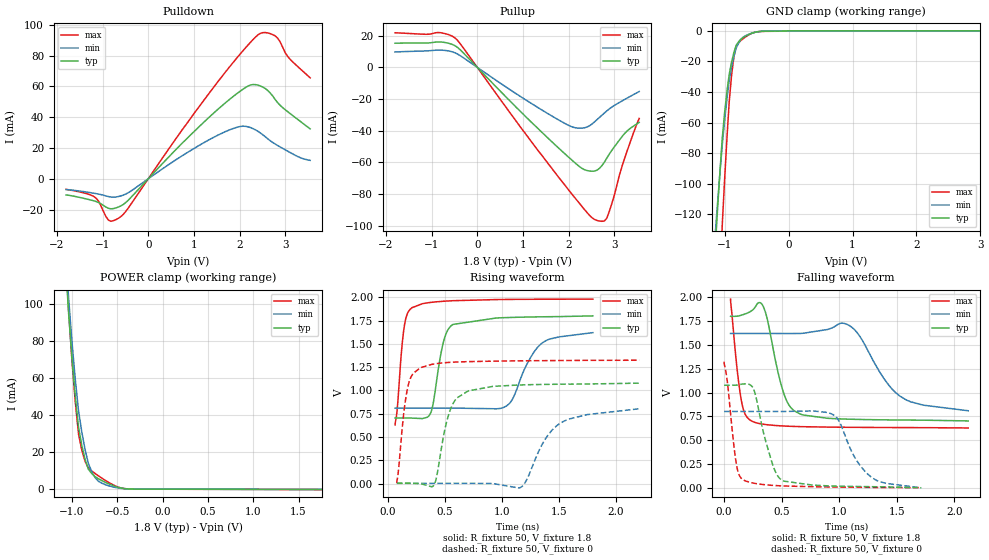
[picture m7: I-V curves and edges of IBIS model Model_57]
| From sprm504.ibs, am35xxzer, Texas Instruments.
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| Model based on original model for BQ1833DV40DTPBFZP18LL_7LM_X50
|   Sub model LL_7LM_X50_PU_ON_1P8
[model]   Model_57
|[Description]  1.8V-I/O-PU-X
|[Input Load]   PU
|[Output Drive]
|Voltage   1.8V
|Mode   I/O
Model_type   I/O
Polarity   Non-Inverting
Enable   Active-Low
Vinl =  0.63V
Vinh =  1.17V
Cref =  15pF
Rref =  100.0000M
Vref =  0V
Vmeas =  0.9
C_comp   2.258279p   2.108893p   2.320297p
[Model Spec]
Vinl   0.63V   0.567V   0.693V
Vinh   1.17V   1.053V   1.287V
[Temperature Range]   25   125   -40
[Voltage Range]   1.8   1.62   1.98
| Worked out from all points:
|   slope of the pulldown table from 0 to 0.27 V, typ, clamps not added: 31.4 ohm
|   slope of the pullup table from 0 to 0.27 V, typ, clamps not added: 33.4 ohm
|   GND clamp passes 1 mA (typ) near -0.53 V on its own axis
|   POWER clamp passes 1 mA (typ) near -0.49 V on its own axis
|   rising waveform, R_fixture 50, V_fixture 1.8: 20-80 % time 96ps typ, 192ps min, 58.1ps max; typ from 0.703 V to 1.8 V
|   rising waveform, R_fixture 50, V_fixture 0: 20-80 % time 125ps typ, 245ps min, 76.8ps max; typ from 0.003 V to 1.08 V
|   falling waveform, R_fixture 50, V_fixture 1.8: 20-80 % time 134ps typ, 277ps min, 76.4ps max; typ from 1.8 V to 0.703 V
|   falling waveform, R_fixture 50, V_fixture 0: 20-80 % time 137ps typ, 213ps min, 71.1ps max; typ from 1.08 V to 0.003 V
[POWER_clamp]
-1.8V     842.3mA    869.2mA    912.6mA
-1.073V   123.5mA    130.8mA    128.8mA
-1.036V   94.69mA    102.8mA    96.31mA
-1V       70.7mA     79.63mA    69.41mA
-963.6mV  50.3mA     59.44mA    47.21mA
-927.3mV  33.48mA    42.27mA    29.73mA
-890.9mV  23.56mA    30.73mA    21mA
-818.2mV  10.72mA    13.8mA     11.42mA
-709.1mV  5.624mA    4.312mA    7.236mA
-527.3mV  1.606mA    1.01mA     1.915mA
-381.8mV  142.3uA    117.5uA    127.8uA
1.764V    -143.5uA   -80.17uA   -225.9uA
[Pulldown]
-1.8V     -10.49mA   -6.992mA   -6.878mA
-1.145V   -14.77mA   -9.642mA   -12.54mA
-872.7mV  -19.18mA   -11.58mA   -26.88mA
-600mV    -17.64mA   -11.15mA   -24.61mA
1.636V    48.04mA    29.95mA    67.37mA
2.073V    58.21mA    34.18mA    83.2mA
2.291V    61.28mA    32.65mA    90.41mA
2.455V    60.33mA    29.78mA    94.55mA
2.618V    57.37mA    25.94mA    94.82mA
2.782V    51.43mA    22.55mA    92.84mA
3.055V    43.59mA    17.92mA    79.47mA
3.545V    32.43mA    11.97mA    65.61mA
[Pullup]
-1.8V     15.27mA    9.71mA     21.85mA
-818.2mV  16.05mA    10.88mA    21.94mA
-490.9mV  13.72mA    9.223mA    18.66mA
1.036V    -30.45mA   -20.11mA   -41.15mA
2.018V    -57.22mA   -36.91mA   -78.08mA
2.345V    -64.63mA   -38.19mA   -89.73mA
2.618V    -65.01mA   -33.11mA   -96.69mA
2.782V    -59.96mA   -28.87mA   -97.07mA
2.836V    -57.32mA   -27.51mA   -95.25mA
3V        -50.25mA   -24.09mA   -80.87mA
3.218V    -42.03mA   -20.43mA   -58.16mA
3.545V    -34.78mA   -15.26mA   -32.29mA
[GND_clamp]
-1.8V     -697.8mA   -553.3mA   -1.259A
-1.145V   -140.7mA   -131.7mA   -248.4mA
-1.109V   -115.2mA   -111.7mA   -203.4mA
-1.036V   -69.7mA    -74.11mA   -126mA
-1V       -53.27mA   -58.3mA    -96.66mA
-927.3mV  -28.09mA   -31.91mA   -45.55mA
-890.9mV  -20.27mA   -23.39mA   -28.66mA
-854.5mV  -14.02mA   -16.45mA   -16.77mA
-818.2mV  -9.337mA   -11.08mA   -9.893mA
-672.7mV  -3.466mA   -3.226mA   -3.973mA
-18.18mV  0A         0A         0A
3.6V      0A         0A         0A
[Ramp]
dV/dt_f  0.7432252/0.14126236n 0.55025481/0.2932849n 0.90207593/80.870476p
dV/dt_r 0.66806868/0.12557629n 0.50965691/0.24625326n 0.81084877/77.361957p
R_load = 50
[Rising Waveform]
R_fixture = 50
V_fixture = 1.8
V_fixture_min = 1.62
V_fixture_max = 1.98
62.46ps   703.3mV    810mV      629.5mV
82.15ps   703.3mV    810mV      808.1mV
140.1ps   703.4mV    810mV      1.66V
210.2ps   702.3mV    810mV      1.888V
373.8ps   756mV      810mV      1.944V
485.7ps   1.515V     810mV      1.957V
569.1ps   1.708V     810mV      1.963V
1.037ns   1.782V     831.3mV    1.977V
1.342ns   1.79V      1.499V     1.979V
1.796ns   1.8V       1.62V      1.98V
[Rising Waveform]
R_fixture = 50
V_fixture = 0
V_fixture_min = 0
V_fixture_max = 0
78.17ps   2.802mV    1.768mV    3.967mV
167.6ps   2.834mV    1.768mV    996.7mV
284.6ps   -815.7uV   1.769mV    1.244V
407.3ps   -8.76mV    1.761mV    1.284V
547.8ps   795.9mV    1.768mV    1.301V
703.6ps   994.3mV    1.79mV     1.309V
1.159ns   1.058V     -43.86mV   1.318V
1.381ns   1.064V     479.9mV    1.32V
1.503ns   1.066V     641.3mV    1.321V
2.202ns   1.078V     802.6mV    1.324V
[Falling Waveform]
R_fixture = 50
V_fixture = 1.8
V_fixture_min = 1.62
V_fixture_max = 1.98
56.23ps   1.8V       1.62V      1.98V
109.3ps   1.801V     1.62V      1.29V
150.4ps   1.812V     1.62V      915.7mV
246.4ps   1.864V     1.62V      698.1mV
340.5ps   1.903V     1.62V      668.9mV
515.9ps   1.002V     1.62V      650.3mV
664.3ps   774.1mV    1.62V      643.5mV
1.067ns   722.3mV    1.716V     636.8mV
1.525ns   713mV      965.4mV    633.7mV
2.121ns   703.3mV    810mV      629.5mV
[Falling Waveform]
R_fixture = 50
V_fixture = 0
V_fixture_min = 0
V_fixture_max = 0
0s        1.078V     802.6mV    1.324V
29ps      1.077V     802.6mV    1.108V
105.9ps   1.079V     802.6mV    258.8mV
163.7ps   1.09V      802.6mV    87.37mV
258ps     1.033V     802.6mV    50.82mV
412.8ps   280.7mV    802.6mV    28.6mV
495.7ps   88.38mV    802.4mV    22.84mV
940.1ps   21.67mV    773.3mV    10.55mV
1.282ns   13.99mV    111.2mV    6.523mV
1.713ns   2.802mV    1.768mV    3.967mV
